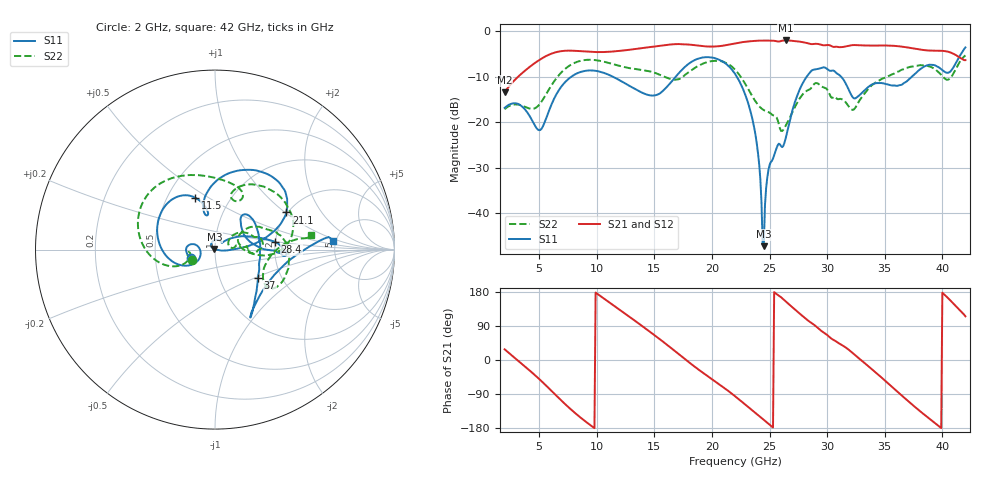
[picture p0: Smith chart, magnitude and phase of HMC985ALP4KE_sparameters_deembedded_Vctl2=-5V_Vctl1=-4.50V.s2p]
!s2p File: Measurements: S11, S21, S12, S22
# GHz S dB R 50.0
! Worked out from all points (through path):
!   401 points, 2 GHz to 42 GHz, reference 50 ohm
!   highest |S21| = -2.06 dB at 26.4 GHz (marker M1); lowest = -13.4 dB at 2 GHz (marker M2)
!   lowest |S11| = -47.2 dB at 24.5 GHz (marker M3), VSWR 1.01, Z = 49.7 + j0.318 ohm
!   |S11| at or under -10 dB: start of sweep to 7.806 GHz; 22.15 GHz to 28.23 GHz (6.083 GHz wide, 24.1 % of centre); 31.2 GHz to 37.36 GHz (6.16 GHz wide, 18 % of centre)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
!   |S22| runs from -21.9 to -5.3 dB; largest |S21 - S12| = 0.0011
!   S11 on the Smith chart (normalised r, x): 2 GHz: 0.76, -0.07; 11.5 GHz: 0.68, +0.44; 21.1 GHz: 1.97, +1.02; 28.4 GHz: 2.00, +0.19; 37 GHz: 1.52, -0.52; 42 GHz: 4.75, +0.84
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2  -16.87 -161.7  -13.43 28.2  -13.44 28.2  -17.17 -155.6
5  -21.77 -172.5  -6.38 -50.1  -6.38 -50.1  -16.18 -159.8
6.3  -14.83 -150.4  -4.76 -88.3  -4.76 -88.3  -11.04 -161.5
8.7  -8.90 150.3  -4.44 -154.5  -4.44 -154.5  -6.47 151.3
11.5  -10.15 111.1  -4.47 143.2  -4.47 143.2  -7.33 105.2
13.6  -13.11 101.2  -3.85 97.2  -3.85 97.2  -8.43 75.8
15.4  -13.81 105.8  -3.25 56.5  -3.25 56.5  -9.52 62.3
17.9  -7.33 80.2  -2.94 -3.5  -2.94 -3.5  -9.18 72.2
21.1  -6.98 27.5  -3.14 -74.3  -3.14 -74.3  -6.87 16.2
22  -9.38 17.0  -2.71 -95.5  -2.71 -95.5  -8.47 0.7
23.6  -20.37 -0.1  -2.18 -135.2  -2.18 -135.2  -14.73 -4.0
24.5  -47.24 132.6  -2.08 -157.9  -2.08 -157.9  -17.36 8.4
25  -29.41 133.3  -2.11 -170.6  -2.11 -170.6  -17.91 11.0
26.4  -23.54 42.5  -2.06 154.7  -2.06 154.7  -20.79 33.1
28.4  -9.42 7.2  -2.73 102.7  -2.73 102.8  -12.90 18.5
28.7  -8.60 2.2  -2.87 96.5  -2.87 96.6  -12.19 16.7
30.7  -8.96 -3.0  -3.45 50.8  -3.45 50.9  -14.47 2.5
32.5  -14.69 32.8  -3.08 10.9  -3.08 10.9  -16.61 28.4
35.4  -11.79 19.2  -3.19 -64.6  -3.18 -64.5  -9.80 19.5
37  -10.84 -33.4  -3.61 -107.7  -3.61 -107.6  -8.02 5.2
39.8  -8.16 -56.9  -4.32 -177.1  -4.32 -177.0  -9.34 -35.0
42  -3.59 4.3  -6.38 115.3  -6.38 115.4  -5.33 8.9
